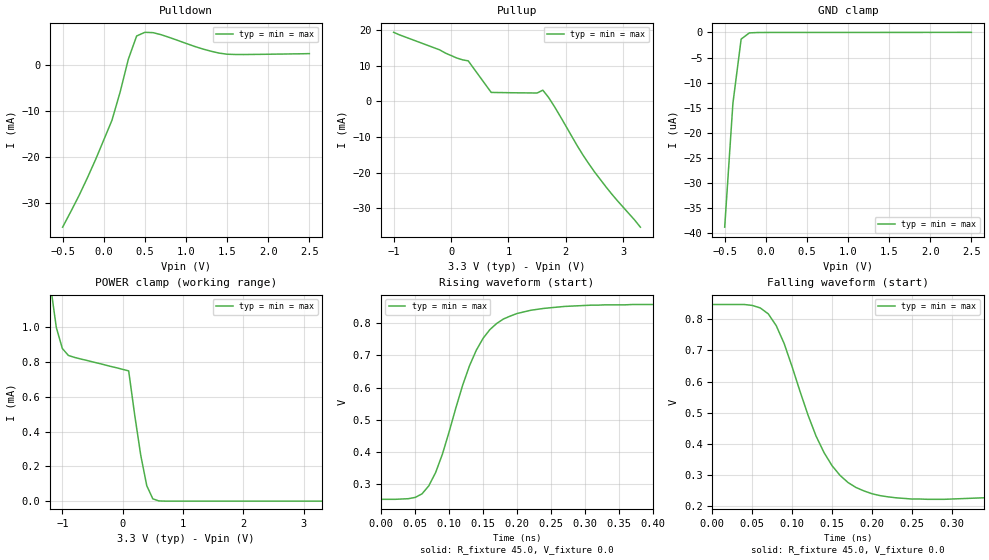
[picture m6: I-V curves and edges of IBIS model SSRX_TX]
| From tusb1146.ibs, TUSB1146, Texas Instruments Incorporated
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[Model] SSRX_TX
Model_type Output
| typ min max
C_comp 0.294p 0.294p 0.284p
[Algorithmic Model]
Executable Windows_cl19.00.24215.1_64  SSRX_TX_x64.dll SSRX_TX.ami
Executable Linux_gcc5.4.0_64 SSRX_TX_x64.so SSRX_TX.ami
[End Algorithmic Model]
[Temperature_Range] 27 27 27
[Voltage Range] 3.3 3.3 3.3
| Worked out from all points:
|   slope of the pulldown table from 0 to 0.495 V, typ, clamps not added: 21.1 ohm
|   slope of the pullup table from 0 to 0.495 V, typ, clamps not added: 85.2 ohm
|   POWER clamp passes 1 mA (typ) near -1.10 V on its own axis
|   rising waveform, R_fixture 45.0, V_fixture 0.0: 20-80 % time 58.3ps typ, 58.3ps min, 58.3ps max; typ from 0.253 V to 0.854 V
|   falling waveform, R_fixture 45.0, V_fixture 0.0: 20-80 % time 51.9ps typ, 51.9ps min, 51.9ps max; typ from 0.848 V to 0.247 V
[GND_clamp]
|   Voltage   I(typ)   I(min)   I(max)
-500mV    -38.8uA    -38.8uA    -38.8uA
-400mV    -14.1uA    -14.1uA    -14.1uA
-300mV    -1.32uA    -1.32uA    -1.32uA
-200mV    -83.7nA    -83.7nA    -83.7nA
-100mV    -11.9nA    -11.9nA    -11.9nA
2.5V      28.8nA     28.8nA     28.8nA
[Power_clamp]
| Note that the[POWER_clamp]voltage table is referenced to Vcc
| and is calculated using Vtable=Vcc - Vmeasured.
|   Voltage   I(typ)   I(min)   I(max)
-1.7V     7.32mA     7.32mA     7.32mA
-1.2V     1.25mA     1.25mA     1.25mA
-1.1V     999uA      999uA      999uA
-1V       878uA      878uA      878uA
-900mV    838uA      838uA      838uA
100mV     749uA      749uA      749uA
200mV     495uA      495uA      495uA
300mV     264uA      264uA      264uA
400mV     88.7uA     88.7uA     88.7uA
500mV     13.4uA     13.4uA     13.4uA
700mV     81.1nA     81.1nA     81.1nA
3.3V      -73.8pA    -73.8pA    -73.8pA
[Pulldown]
|   Voltage   I(typ)   I(min)   I(max)
-500mV    -35.3mA    -35.3mA    -35.3mA
-300mV    -28.4mA    -28.4mA    -28.4mA
-200mV    -24.6mA    -24.6mA    -24.6mA
100mV     -12mA      -12mA      -12mA
200mV     -5.81mA    -5.81mA    -5.81mA
300mV     1.36mA     1.36mA     1.36mA
400mV     6.37mA     6.37mA     6.37mA
500mV     7.17mA     7.17mA     7.17mA
600mV     7.1mA      7.1mA      7.1mA
1.2V      3.56mA     3.56mA     3.56mA
1.5V      2.4mA      2.4mA      2.4mA
2.5V      2.53mA     2.53mA     2.53mA
[Pullup]
|   Voltage   I(typ)   I(min)   I(max)
| Note that the[Pullup]voltage table is referenced to Vcc
| and is calculated using Vtable=Vcc - Vmeasured.
-1V       19.3mA     19.3mA     19.3mA
-200mV    14.4mA     14.4mA     14.4mA
100mV     12.1mA     12.1mA     12.1mA
300mV     11.3mA     11.3mA     11.3mA
700mV     2.46mA     2.46mA     2.46mA
1.5V      2.29mA     2.29mA     2.29mA
1.6V      3.09mA     3.09mA     3.09mA
1.8V      -1.46mA    -1.46mA    -1.46mA
2.2V      -12.5mA    -12.5mA    -12.5mA
2.5V      -19.8mA    -19.8mA    -19.8mA
2.8V      -26mA      -26mA      -26mA
3.3V      -35.3mA    -35.3mA    -35.3mA
[Ramp]
|   typ   min   max
dV/dt_r   0.36/59p 0.36/59p 0.36/59p
dV/dt_f   0.36/46p 0.36/46p 0.36/46p
R_load = 45ohm | Note: Measurement is single ended with 25ohm to ground
[Rising Waveform]
R_fixture = 45.0
V_fixture = 0.0
V_fixture_min = 0.0
V_fixture_max = -0.0
C_fixture = 0p
L_fixture = 0n
|   V(typ)   V(min)   V(max)
0s        253mV      253mV      253mV
50ps      259mV      259mV      259mV
70ps      295mV      295mV      295mV
90ps      393mV      393mV      393mV
130ps     668mV      668mV      668mV
140ps     716mV      716mV      716mV
160ps     780mV      780mV      780mV
200ps     830mV      830mV      830mV
310ps     856mV      856mV      856mV
9.9ns     854mV      854mV      854mV
[Falling Waveform]
R_fixture = 45.0
V_fixture = 0.0
V_fixture_min = 0.0
V_fixture_max = -0.0
C_fixture = 0p
L_fixture = 0n
|   V(typ)   V(min)   V(max)
0s        848mV      848mV      848mV
50ps      845mV      845mV      845mV
70ps      818mV      818mV      818mV
90ps      722mV      722mV      722mV
130ps     424mV      424mV      424mV
160ps     298mV      298mV      298mV
200ps     239mV      239mV      239mV
250ps     222mV      222mV      222mV
740ps     244mV      244mV      244mV
9.9ns     247mV      247mV      247mV
